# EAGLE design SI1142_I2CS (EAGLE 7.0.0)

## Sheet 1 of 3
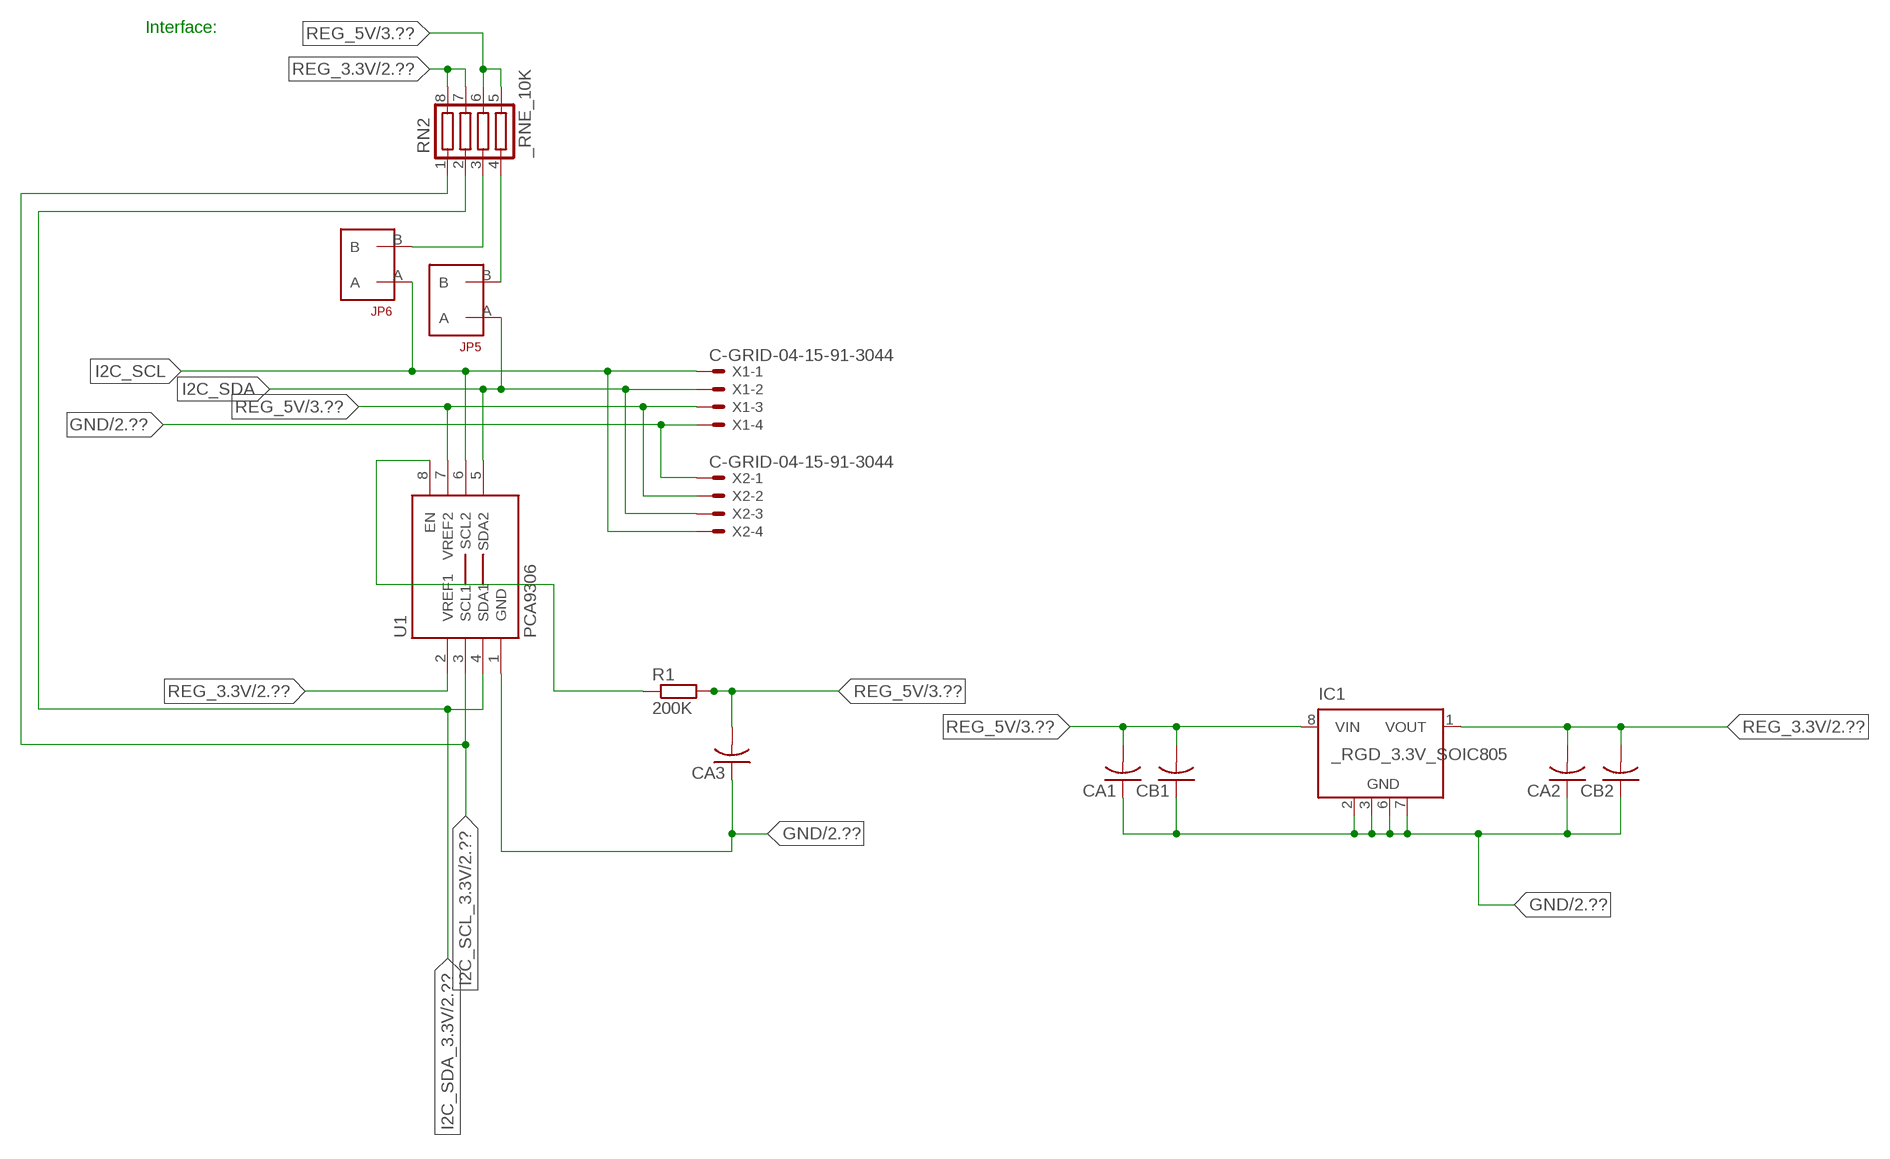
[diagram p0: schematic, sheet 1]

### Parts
CA1  CC1206KRX7R9BB104  [.1UF]
CA2  CC1206KRX7R9BB104  [.1UF]
CA3  CC1206KRX7R9BB104  [.1UF]
CB1  TMK316F106ZL-TC1206K  [TMK316F106ZL-T]
CB2  TMK316F106ZL-TC1206K  [TMK316F106ZL-T]
IC1  _RGD_3.3V_SOIC805  [_RGC_3.3V_SOIC8]
JP5  JUMPER_1X2_2MM  [JUMPER_1X2_2MM]
JP6  JUMPER_1X2_2MM  [JUMPER_1X2_2MM]
R1  200K  RESISTOR_SMT-0603  [R603]
RN2  _RNE_10K  [RNE]
U1  PCA9306  PCA9306_NCD  [PSOP-8]
X1  C-GRID-04-15-91-3044  [15-91-04]
X2  C-GRID-04-15-91-3044  [15-91-04]

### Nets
GND: CA1.1 CA2.1 CA3.1 CB1.1 CB2.1 IC1.2(GND) IC1.3(GND) IC1.6(GND) IC1.7(GND) U1.1(GND) X1.4 X2.1 ; also sheet 2,3
I2C_SCL: JP6.A U1.6(SCL2) X1.1 X2.4
I2C_SCL_3.3V: RN2.1 U1.3(SCL1) ; also sheet 2
I2C_SDA: JP5.A U1.5(SDA2) X1.2 X2.3
I2C_SDA_3.3V: RN2.2 U1.4(SDA1) ; also sheet 2
N$1: JP6.B RN2.3
N$2: JP5.B RN2.4
N$3: R1.1 U1.8(EN)
REG_3.3V: CA2.2 CB2.2 IC1.1(VOUT) RN2.7 RN2.8 U1.2(VREF1) ; also sheet 2
REG_5V: CA1.2 CA3.2 CB1.2 IC1.8(VIN) R1.2 RN2.5 RN2.6 U1.7(VREF2) X1.3 X2.2 ; also sheet 3
Unconnected: IC1.4(NC) IC1.5(NC)

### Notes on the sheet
- Interface:

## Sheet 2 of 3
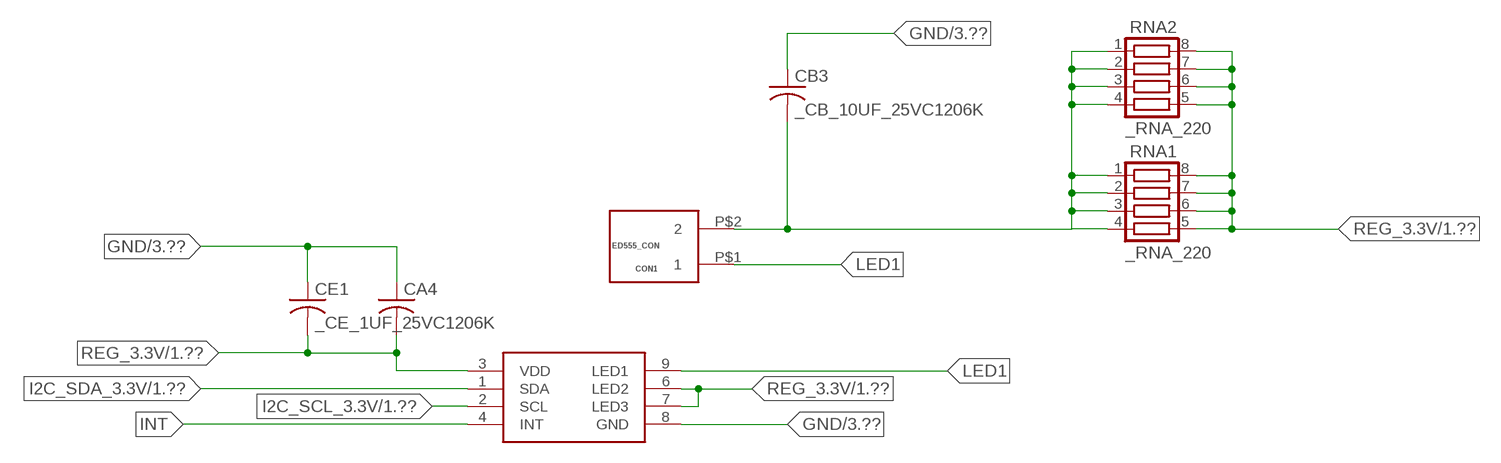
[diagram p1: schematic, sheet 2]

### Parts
CA4  _CA_.10UF_50VC1206K  [_CA_.1UF_50V]
CB3  _CB_10UF_25VC1206K  [_CB_10UF_25V]
CE1  _CE_1UF_25VC1206K  [CE]
CON1  ED555_CON  [ED555_CON]
IC2  SI1142  SI1145  [SI1145]
RNA1  _RNA_220  [RNA]
RNA2  _RNA_220  [RNA]

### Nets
GND: CA4.1 CB3.1 CE1.1 IC2.8(GND) ; also sheet 1,3
I2C_SCL_3.3V: IC2.2(SCL) ; also sheet 1
I2C_SDA_3.3V: IC2.1(SDA) ; also sheet 1
INT: IC2.4(INT)
LED1: CON1.P$1 IC2.9(LED1)
N$11: CB3.2 CON1.P$2 RNA1.1 RNA1.2 RNA1.3 RNA1.4 RNA2.1 RNA2.2 RNA2.3 RNA2.4
REG_3.3V: CA4.2 CE1.2 IC2.3(VDD) IC2.6(LED2) IC2.7(LED3) RNA1.5 RNA1.6 RNA1.7 RNA1.8 RNA2.5 RNA2.6 RNA2.7 RNA2.8 ; also sheet 1

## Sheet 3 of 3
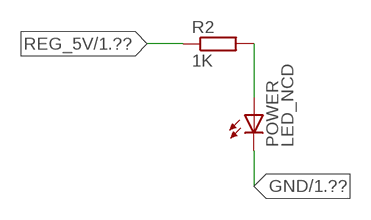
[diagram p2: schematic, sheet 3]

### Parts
POWER  LED_NCD  [CHIPLED_0603]
R2  1K  RESISTOR_SMT-0402  [R402]

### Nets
GND: POWER.C ; also sheet 1,2
N$4: POWER.A R2.2
REG_5V: R2.1 ; also sheet 1

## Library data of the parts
CA1-CA3 = NCD_ULTIMATE_LIBRARY:CC1206KRX7R9BB104: Capacitor CA .1uF 50V SMT C1206K CC1206KRX7R9BB104
CA4 = NCD_ULTIMATE_LIBRARY:_CA_.10UF_50V: Capacitor .1uF SMT
CB1 CB2 = NCD_ULTIMATE_LIBRARY:TMK316F106ZL-T: Capacitor CB 10uF SMT 1206 TMK316F106ZL-T
CB3 = NCD_ULTIMATE_LIBRARY:_CB_10UF_25V: Capacitor 10uF SMT
CE1 = NCD_ULTIMATE_LIBRARY:_CE_1UF_25V: Capacitor 1uF SMT
CON1 = NCD_ULTIMATE_bhaskar:ED555_CON: Digikey ED1514-ND/ ED555/2DS NCD CON
IC1 = NCD_ULTIMATE_LIBRARY:_RGD_3.3V_SOIC8: Regulator Linear 3.3V Chip Positive VOLTAGE REGULATOR Digikey 497-1199-2-ND/L78L33ACD13TR
IC2 = NCD_ULTIMATE_bhaskar:SI1145: Digikey 336-2200-6-ND/SI1142-A11-GMR
JP5 JP6 = NCD_ULTIMATE_CONNECTORS:JUMPER_1X2_2MM
POWER = NCD_ULTIMATE_LIBRARY:LED_NCD: LED Digikey 754-1132-2-ND/APT2012SRCPRV
R1 R2 = NCD_ULTIMATE_LIBRARY:RESISTOR_SMT: NCD Resistor
RN2 = NCD_ULTIMATE_LIBRARY:_RNE_10K: Resistor Array RNE SMT 10K x 4 Single Resistor Source: http://www.ctscorp.com/components/Datasheets/CTSChipArrayDs.pdf Digikey 742C083103JPTR-ND/742C083103JP; OC_FARNELL: unknown; OC_NEWARK: unknown
RNA1 RNA2 = NCD_ULTIMATE_LIBRARY:_RNA_220: Resistor Array RNA SMT 220 x 4 Single Resistor Source: http://www.ctscorp.com/components/Datasheets/CTSChipArrayDs.pdf Digikey 742C083221JPTR-ND/742C083221JP; OC_FARNELL: unknown; OC_NEWARK: unknown
U1 = NCD_ULTIMATE_LIBRARY:PCA9306_NCD: NCD Bidirectional I2C level shifter. NOT compatible with all available part number pinout schemes- DOUBLE CHECK!!!; PROD_ID: IC-10023
X1 X2 = NCD_ULTIMATE_CONNECTORS:C-GRID-04: CONNECTOR 4-Pos I2C wire to board 2.54 mm (0.100") pitch header Digikey WM1342-ND/0015912045; OC_FARNELL: unknown; OC_NEWARK: unknown

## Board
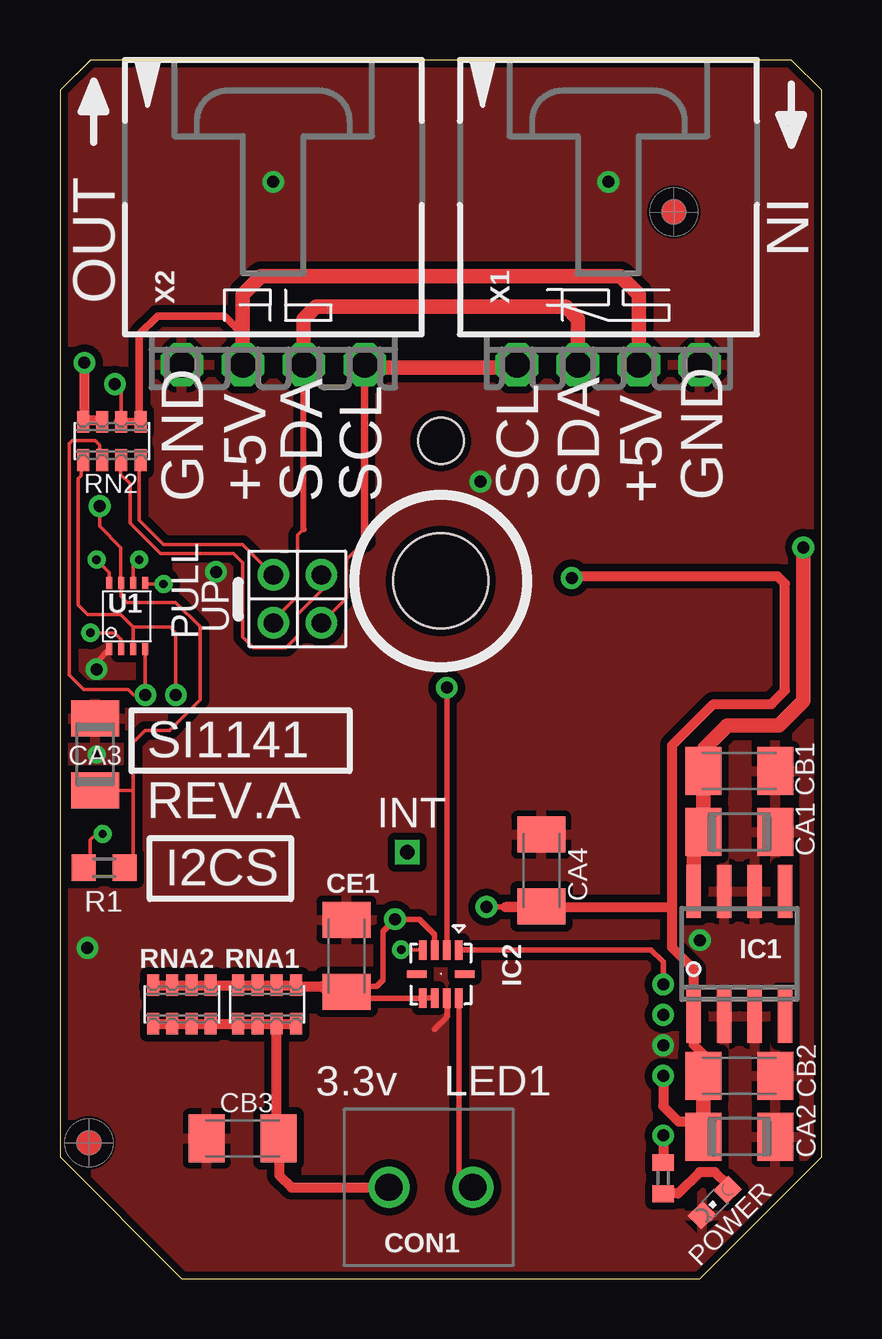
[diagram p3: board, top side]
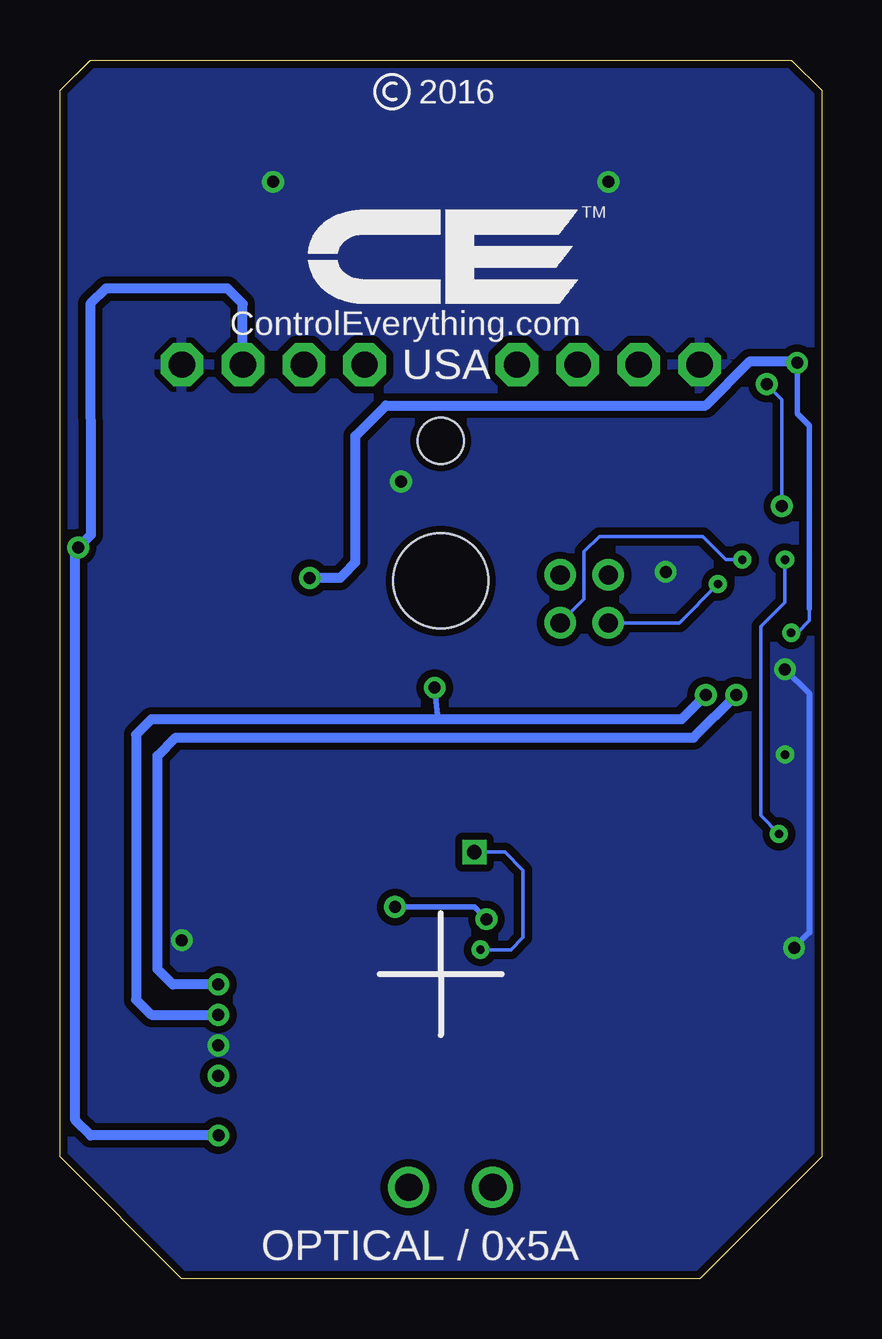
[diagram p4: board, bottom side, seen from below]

Size 31.75 x 50.8 mm. Coordinates in mm from the lower left corner, seen from the top.
Outline: 48 segments
Copper layers (1*16): Top 0.035mm / dielectric 1.5mm / Bottom 0.035mm
Design rules "default": minimum track width 5mil, minimum drill 24mil, track to track 5mil, track to pad 5mil, pad to pad 5mil, via to via 5mil, smd to smd 5mil, copper to edge 10mil, drill to drill 8mil, minimum pad ring 10mil, minimum via ring 8mil, stop-mask expansion 2mil, vias tented up to drill 0mil, thermal gap 10mil
Holes 3.96 mm at 15.88,29.08
Holes 1.91 mm at 15.88,34.93

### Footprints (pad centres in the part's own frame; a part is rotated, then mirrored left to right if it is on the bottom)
.1UF = smd 1.5 x 2: 1 -1.5,0; 2 1.5,0
_CA_.1UF_50V = smd 1.5 x 2: 1 -1.5,0; 2 1.5,0
TMK316F106ZL-T = smd 1.5 x 2: 1 -1.5,0; 2 1.5,0
_CB_10UF_25V = smd 1.5 x 2: 1 -1.5,0; 2 1.5,0
CE = smd 1.5 x 2: 1 -1.5,0; 2 1.5,0
ED555_CON = drill 1.143: P$1 0,3.5; P$2 0,0
_RGC_3.3V_SOIC8 = smd 0.6 x 2.2: 1 -1.905,-2.6; 2 -0.635,-2.6; 3 0.635,-2.6; 4 1.905,-2.6; 5 1.905,2.6; 6 0.635,2.6; 7 -0.635,2.6; 8 -1.905,2.6
SI1145 = smd 0.8 x 0.3: 1 -1,0.75; 2 -1,0.25; 3 -1,-0.25; 4 -1,-0.75; 6 1,-0.75; 7 1,-0.25; 8 1,0.25; 9 1,0.75 | smd 0.3 x 0.8: 5 0,-1; 10 0,1
JUMPER_1X2_2MM = drill 0.8: A 0,2; B 0,0
CHIPLED_0603 = smd 0.8 x 0.876: A 0,-0.75; C 0,0.75
R603 = smd 1 x 1.1: 1 -0.85,0; 2 0.85,0
R402 = smd 0.7 x 0.9: 1 -0.65,0; 2 0.65,0
RNE = smd 0.5 x 0.9: 1 -1.2,-0.8; 2 -0.4,-0.8; 3 0.4,-0.8; 4 1.2,-0.8; 5 1.2,0.8; 6 0.4,0.8; 7 -0.4,0.8; 8 -1.2,0.8
RNA = smd 0.5 x 0.9: 1 -1.2,-0.8; 2 -0.4,-0.8; 3 0.4,-0.8; 4 1.2,-0.8; 5 1.2,0.8; 6 0.4,0.8; 7 -0.4,0.8; 8 -1.2,0.8
PSOP-8 = smd 0.25 x 0.5: 1 -0.73,-1.37; 2 -0.23,-1.37; 3 0.27,-1.37; 4 0.77,-1.37; 5 0.77,1.38; 6 0.27,1.38; 7 -0.23,1.38; 8 -0.73,1.38
15-91-04 = drill 1.1 pad 1.778 octagon: 1 -3.81,-7.62; 2 -1.27,-7.62; 3 1.27,-7.62; 4 3.81,-7.62

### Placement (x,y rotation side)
CA1  28.32,18.62 180 top
CA2  28.32,5.92 180 top
CA3  1.46,21.86 270 top
CA4  20.07,17.02 270 top
CB1  28.32,21.16 180 top
CB2  28.32,8.46 180 top
CB3  7.62,5.84 0 top
CE1  11.94,13.46 270 top
CON1  13.72,3.81 270 top
IC1  28.32,13.54 0 top
IC2  15.88,12.7 270 top
JP5  8.89,29.34 180 top
JP6  10.9,29.34 180 top
POWER  27.3,3.18 135 top
R1  1.84,17.13 0 top
R2  25.15,4.19 270 top
RN2  2.16,34.93 0 top
RNA1  8.64,11.43 0 top
RNA2  5.08,11.43 0 top
U1  2.79,27.61 0 top
U$5  [VISION_REF10]  1.21,5.66 90 top
U$28  [VISION_REF10]  25.59,44.46 90 top
X1  22.86,45.72 0 top
X2  8.89,45.72 0 top

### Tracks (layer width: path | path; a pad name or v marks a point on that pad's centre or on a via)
GND  (via drill 0.35, 0.5)
  Top 0.152: CA3.1 1.52,23.42 1.52,23.62
  Top 0.254: IC2.8 16.12,10.92 15.62,10.41 | v1.52,25.4 1.52,25.7 U1.1
  Bottom 0.254: v1.52,25.4 0.51,24.38 0.51,14.43 v1.15,13.79
  other vias: 8.89,45.72 22.86,45.72 25.15,9.73 17.53,33.22 26.67,14.11 6.5,29.46 1.52,21.84
  pour Bottom (isolate 0.305): -0.64,5.08 -0.64,49.53 1.27,51.44 30.48,51.44 32.38,49.53 32.38,5.08 26.67,-0.63 5.08,-0.63
  pour Top (isolate 0.305): 4.45,-1.27 -1.27,4.45 -1.27,50.17 0.64,52.07 31.11,52.07 33.02,50.17 33.02,4.45 27.3,-1.27
I2C_SCL  (via drill 0.35)
  Top 0.152: 12.7,30.73 11.94,29.97 11.94,28.38 JP6.A | v3.3,29.97 3.06,29.96 U1.6
  Top 0.305: 12.7,30.73 X2.4
  Top 0.406: X2.4 12.7,37.97 | 19.05,37.97 X1.1
  Top 0.61: 12.7,37.97 19.05,37.97
  Bottom 0.152: JP6.A 9.91,28.33 9.91,30.3 9.27,30.94 4.96,30.94 3.99,29.97 v3.3,29.97
I2C_SCL_3.3V  (via drill 0.5)
  Top 0.152: RN2.1 0.89,34.07 0.89,33.48 0.77,33.35 0.77,28.08 1.16,27.69 2.54,27.69 3.06,27.17 | 3.06,27.17 U1.3 | v4.83,24.33 v4.83,24.34 4.83,26.92 4.58,27.17 3.06,27.17
  Top 0.229: IC2.2 v16.13,24.64
  Bottom 0.229: v16.13,24.64 16,23.32
  Bottom 0.406: v4.83,24.33 5.84,23.32 16,23.32 27.94,23.32 28.58,22.68 28.58,11.63 27.94,11 v25.15,11
I2C_SDA  (via drill 0.35)
  Top 0.152: JP5.A 8.89,27.44 9.91,28.45 9.91,30.99 10.16,31.24 | U1.5 3.6,28.96 v4.32,28.96
  Top 0.254: 10.16,31.24 10.16,31.25 X2.3
  Top 0.61: X2.3 10.16,40.01 10.67,40.51 21.09,40.51 21.59,40.01 X1.2
  Bottom 0.152: v4.32,28.96 5.94,27.34 JP5.A
I2C_SDA_3.3V  (via drill 0.5)
  Top 0.152: RN2.2 1.65,34.14 1.65,34.75 1.46,34.94 0.51,34.94 0.38,34.81 0.38,26.37 0.38,26.36 0.38,25.17 0.99,24.56 2.85,24.56 3.07,24.33 v3.56,24.33 v3.56,24.34 U1.4
  Top 0.229: IC2.1 16.64,13.72 24.64,13.72 25.15,13.21 v25.15,12.27
  Bottom 0.406: v25.15,12.27 27.05,12.27 27.69,12.9 27.69,21.79 26.93,22.56 5.34,22.56 v3.56,24.33
INT  (via drill 0.35, 0.6)
  Top 0.152: IC2.4 14.98,13.72 v14.22,13.72
  Bottom 0.152: v14.22,13.72 12.95,13.72 12.45,14.22 12.45,17.02 13.21,17.78 v14.48,17.78
LED1
  Top 0.229: IC2.9 16.64,11.56 16.64,4.19 17.02,3.81 CON1.P$1
N$1
  Top 0.152: JP6.B 10.92,29.31 10.92,28.7 9.91,27.69 9.91,26.8 9.42,26.31 8.06,26.31 7.62,26.75 7.62,29.84 7.24,30.23 4.19,30.23 2.92,31.5 2.92,33.15 2.54,33.53 2.54,34.1 RN2.3
  Top 0.305: 2.54,34.02 RN2.3
N$2
  Top 0.152: JP5.B 7.62,30.61 4.32,30.61 3.3,31.62 3.3,34.07 RN2.4
  Top 0.305: 3.37,33.88 RN2.4
N$3  (via drill 0.35)
  Top 0.152: R1.1 1.27,17.41 1.27,18.29 1.52,18.54 v1.78,18.54 | v1.52,29.97 2.06,29.44 U1.8
  Bottom 0.152: v1.78,18.54 2.54,19.3 2.54,27.18 1.52,28.19 v1.52,29.97
N$4
  Top 0.406: POWER.A 27.84,3.92 27.3,4.45 26.67,4.45 25.78,3.56 25.16,3.56 R2.2
N$11
  Top 0.406: RNA2.1 RNA2.2 RNA2.3 RNA2.4 RNA1.1 RNA1.2 RNA1.3 | RNA1.3 RNA1.4 | RNA1.3 9.04,5.93 CB3.2 9.14,5.82 9.14,4.32 9.65,3.81 CON1.P$2
REG_3.3V  (via drill 0.35, 0.5)
  Top 0.152: v1.27,26.92 2.29,26.92 2.56,26.65 U1.2
  Top 0.229: CE1.2 12.17,12.19 | IC2.7 IC2.6 14.98,11.68 12.45,11.68 12.17,11.96 CE1.2 | CA4.2 18.52,15.49 v17.78,15.49 | CE1.2 12.22,11.96 12.45,12.19 13.21,12.19 13.46,12.45 13.46,14.48 v13.97,14.99 14.99,14.99 15.62,14.35 IC2.3
  Top 0.406: CB2.2 26.82,9.35 26.42,9.75 26.42,10.36 | v25.15,8.46 25.15,7.19 25.78,6.55 26.82,6.55 | IC1.1 26.42,12.9 25.53,13.79 25.53,15.49 | 25.53,15.49 25.53,22.24 27.24,23.95 29.66,23.95 30.23,24.52 30.23,28.97 29.91,29.29 21.41,29.29 v21.34,29.21 | 26.52,5.62 CA2.2 | v1.02,38.18 1.02,35.78 | 1.02,35.78 RN2.8 | 1.02,35.78 1.71,35.78 RN2.7 | RNA2.8 3.84,12.19 3.81,12.19 3.85,12.23 RNA2.7 RNA2.6 RNA2.5 RNA1.8 RNA1.7 RNA1.6 RNA1.5 9.87,12.19 10.92,12.19 11.15,11.96 CE1.2 | CA4.2 18.57,15.49 25.53,15.49
  Top 0.61: CB2.2 26.82,6.55 CA2.2 | 26.42,10.36 IC1.1
  Bottom 0.152: 0.51,27.94 0.51,27.43 1.02,26.92 v1.27,26.92
  Bottom 0.229: 0.51,27.94 0.51,35.56 1.02,36.07 v1.02,38.18 | v17.78,15.49 14.48,15.49 v13.97,14.99
  Bottom 0.406: v1.02,38.18 1.08,38.24 2.99,38.24 4.83,36.4 18.16,36.4 19.43,35.13 19.43,29.87 19.94,29.34 20.07,29.21 v21.34,29.21
REG_5V  (via drill 0.5)
  Top 0.152: RN2.6 2.56,37.01 v2.29,37.29 | R1.2 3.05,17.49 3.05,20.36 | 3.05,20.36 3.05,22.35 3.56,22.86 4.57,22.86 5.84,24.13 5.84,27.18 4.83,28.19 2.79,28.19 2.56,28.43 U1.7 2.54,29.01 2.54,30.48 1.65,31.37 v1.65,32.21 | CA3.2 3.05,20.36
  Top 0.305: 7.62,39.37 7.5,39.37 | 2.42,35.74 RN2.6 RN2.5 3.31,35.8 3.31,39.37 4.07,40.13 6.86,40.13 7.62,39.37 | X2.2 7.62,39.37
  Top 0.406: v25.15,5.97 R2.1
  Top 0.61: X1.3 24.13,41.02 23.37,41.78 8.38,41.78 7.62,41.02 X2.2 | IC1.8 26.42,18.21 CA1.2 CB1.2 26.86,21.2 26.86,22.11 27.82,23.06 29.98,23.06 30.99,24.08 v30.99,30.48
  Bottom 0.152: v1.65,32.21 1.65,36.65 v2.29,37.29
  Bottom 0.406: X1.3 24.13,40.64 24.77,41.28 29.84,41.28 30.48,40.64 30.47,31 v30.99,30.48 31.11,30.36 31.11,6.6 30.48,5.97 v25.15,5.97

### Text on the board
tNames: IN | OUT | GND | +5V | SDA | SCL | SCL | SDA | +5V | GND | PULL | UP | SI1141 | REV.A | INT | I2CS | 3.3v | LED1
bNames: 2016 | TM | ControlEverything.com | USA | OPTICAL / 0x5A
